FUNCTION_BLOCK FB_EnableAxes
VAR_INPUT
	bEnableAxes: BOOL:= TRUE;
END_VAR
VAR_OUTPUT
	bAllAxesReady:	BOOL:= FALSE;
END_VAR
VAR_IN_OUT
	stX:	AXIS_REF;
	stY:	AXIS_REF;
	stZ:	AXIS_REF;
	stM1:	AXIS_REF;
	stM2:	AXIS_REF;
	stM3:	AXIS_REF;
END_VAR
VAR
	fOverride:	LREAL	:= 100.0;
	fbPowerX:	MC_Power;
	fbPowerY:	MC_Power;
	fbPowerZ:	MC_Power;
	fbPowerM1:	MC_Power;
	fbPowerM2:	MC_Power;
	fbPowerM3:	MC_Power;
END_VAR

stX.ReadStatus();
stY.ReadStatus();
stZ.ReadStatus();
stM1.ReadStatus();
stM2.ReadStatus();
stM3.ReadStatus();


fbPowerX(
	Enable:=bEnableAxes, 
	Enable_Positive:=bEnableAxes, 
	Enable_Negative:=bEnableAxes, 
	Override:=fOverride, 
	BufferMode:= , 
	Axis:=stX, 
	Status=> , 
	Busy=> , 
	Active=> , 
	Error=> , 
	ErrorID=> );
fbPowerY(
	Enable:=bEnableAxes, 
	Enable_Positive:=bEnableAxes, 
	Enable_Negative:=bEnableAxes, 
	Override:=fOverride, 
	BufferMode:= , 
	Axis:=stY, 
	Status=> , 
	Busy=> , 
	Active=> , 
	Error=> , 
	ErrorID=> );	
fbPowerZ(
	Enable:=bEnableAxes, 
	Enable_Positive:=bEnableAxes, 
	Enable_Negative:=bEnableAxes, 
	Override:=fOverride, 
	BufferMode:= , 
	Axis:=stZ, 
	Status=> , 
	Busy=> , 
	Active=> , 
	Error=> , 
	ErrorID=> );	
fbPowerM1(
	Enable:=bEnableAxes, 
	Enable_Positive:=bEnableAxes, 
	Enable_Negative:=bEnableAxes, 
	Override:=fOverride, 
	BufferMode:= , 
	Axis:=stM1, 
	Status=> , 
	Busy=> , 
	Active=> , 
	Error=> , 
	ErrorID=> );	
fbPowerM2(
	Enable:=bEnableAxes, 
	Enable_Positive:=bEnableAxes, 
	Enable_Negative:=bEnableAxes, 
	Override:=fOverride, 
	BufferMode:= , 
	Axis:=stM2, 
	Status=> , 
	Busy=> , 
	Active=> , 
	Error=> , 
	ErrorID=> );	
fbPowerM3(
	Enable:=bEnableAxes, 
	Enable_Positive:=bEnableAxes, 
	Enable_Negative:=bEnableAxes, 
	Override:=fOverride, 
	BufferMode:= , 
	Axis:=stM3, 
	Status=> , 
	Busy=> , 
	Active=> , 
	Error=> , 
	ErrorID=> );	
bAllAxesReady	:= fbPowerX.Status AND fbPowerY.Status AND fbPowerZ.Status AND 
	fbPowerM1.Status AND fbPowerM2.Status AND fbPowerM3.Status;

END_FUNCTION_BLOCK
